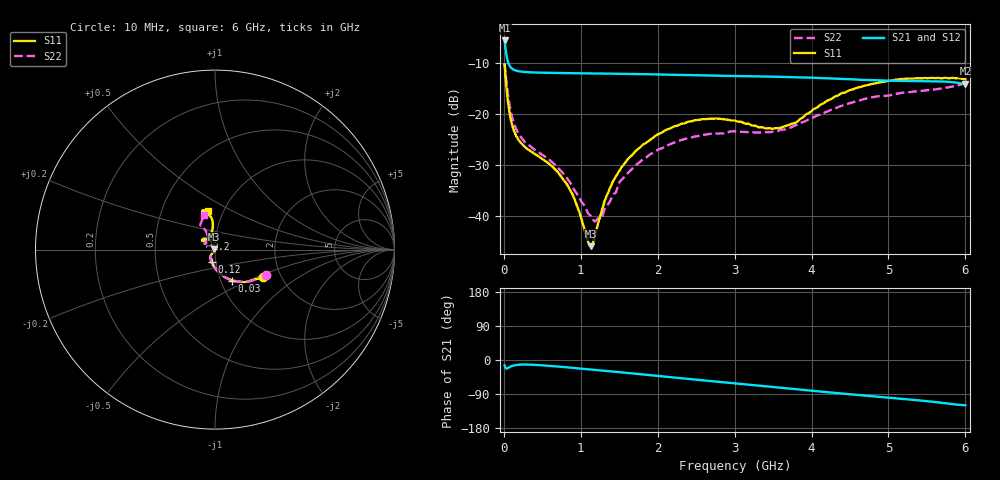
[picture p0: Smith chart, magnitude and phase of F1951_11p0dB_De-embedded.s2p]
! Integrated Device Technology
! Corporate Headquarters
! 6024 Silver Creek Valley Road
! San Jose, CA 95138  USA
! Phone:  1-408-284-8200
! Toll Free:  1-800-223-1366
! Webpage:  http://www.idt.com/
! Timing and RF Division
! 515 Groton Road, Suite 102
! Westford, MA 01886-6024
! Device:  F1951
! Description: 6-bit 0.5 dB Digital Step Attenuator
! Frequency:  100.0 -  4000.00 MHz
! Package:  4x4 mm Thin QFN Plastic Package: 24 pin
! Ports:  2 RF, 6 DC
!  Pin  1  = NC
!  Pin  2  = RF1  =  Port 1
!  Pin  3  = GND
!  Pin  4  = NC
!  Pin  5  = Serial Data Out (SDO)
!  Pin  6  = NC
!  Pin  7  = Reset Bar ( RSTb)
!  Pin  8  = Clock (CLK)
!  Pin  9  = Chip Select Bar (CSb)
!  Pin 10  = NC
!  Pin 11  = Serial Data In (SDI)
!  Pin 12  = NC
!  Pin 13  = NC
!  Pin 14  = VDD
!  Pin 15  = NC
!  Pin 16  = GND
!  Pin 17  = RF2  =  Port 2
!  Pin 18  = NC
!  Pin 19  = GND
!  Pin 20  = GND
!  Pin 21  = GND
!  Pin 22  = GND
!  Pin 23  = GND
!  Pin 24  = GND
! State:  22
! Atten State:  11.0 dB
! Voltage:  +3.30 Volts
! Current:  0.474 mA
! Data:  The device was measured on a F195X evaluation board which has
!  individual transmission lines to the RF pins.  Data was collected
!  de-embedded using a Automatic Fixture Removal [AFR] (Keysight Technologies).
!  The reference plane is the edge of the package pin.
! Misc:  Lot Code  1225BCA
!  Action Tracker AT0399
! Date Measured:  2018-09-13
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# GHz S dB R 50
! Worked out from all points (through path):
!   600 points, 10 MHz to 6 GHz, reference 50 ohm
!   highest |S21| = -5.51 dB at 10 MHz (marker M1); lowest = -14.0 dB at 6 GHz (marker M2)
!   group delay of S21, straight-line fit = 52.2 ps
!   lowest |S11| = -45.9 dB at 1.13 GHz (marker M3), VSWR 1.01, Z = 49.5 + j0.0747 ohm
!   |S11| at or under -10 dB: start of sweep to end of sweep
!   |S22| runs from -41.0 to -10.0 dB; largest |S21 - S12| = 0.00045
!   S11 on the Smith chart (normalised r, x): 10 MHz: 1.61, -0.55; 30 MHz: 1.13, -0.41; 120 MHz: 0.96, -0.14; 2.2 GHz: 0.91, +0.11; 6 GHz: 0.85, +0.39
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0.01  -10.24 -30.3  -5.51 -14.6  -5.51 -14.6  -9.96 -26.2
0.03  -14.06 -60.9  -7.98 -22.4  -7.98 -22.4  -13.09 -54.1
0.07  -19.31 -87.2  -10.34 -19.2  -10.34 -19.2  -17.84 -81.4
0.12  -22.74 -103.1  -11.18 -15.0  -11.19 -15.0  -21.21 -98.3
0.27  -26.36 -122.1  -11.69 -11.9  -11.69 -11.9  -25.42 -120.1
0.79  -33.11 -124.9  -11.90 -18.8  -11.91 -18.8  -31.91 -130.3
0.9  -35.95 -125.4  -11.94 -20.8  -11.94 -20.8  -34.42 -132.4
1.01  -40.62 -133.7  -11.96 -22.8  -11.97 -22.8  -37.18 -138.2
1.13  -45.89 171.5  -11.98 -24.9  -11.98 -24.9  -39.89 -159.4
1.26  -39.53 115.3  -12.00 -27.4  -12.00 -27.4  -40.35 160.9
1.38  -34.47 106.8  -12.02 -29.8  -12.02 -29.8  -37.07 136.1
1.49  -31.39 106.8  -12.06 -31.8  -12.06 -31.8  -33.64 131.0
1.72  -27.11 111.7  -12.10 -36.4  -12.10 -36.4  -29.91 125.4
2.01  -23.88 121.1  -12.18 -42.2  -12.19 -42.2  -26.90 131.2
2.2  -22.46 126.9  -12.24 -46.0  -12.24 -46.0  -25.63 135.9
2.59  -20.94 138.7  -12.36 -53.7  -12.36 -53.7  -24.04 145.7
3.01  -21.26 145.4  -12.50 -61.8  -12.50 -61.8  -23.32 149.4
3.57  -22.72 122.5  -12.63 -72.7  -12.64 -72.7  -23.22 131.4
4.01  -19.20 97.7  -12.82 -81.3  -12.82 -81.3  -20.74 117.8
4.49  -15.29 95.9  -13.11 -90.2  -13.12 -90.2  -17.85 117.0
5.01  -13.44 104.4  -13.40 -99.2  -13.41 -99.2  -16.30 120.4
6  -13.11 99.8  -14.02 -119.3  -14.02 -119.3  -13.91 107.5
